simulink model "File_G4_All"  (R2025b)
settings: Solver=FixedStepDiscrete  StartTime=0.0  StopTime=inf  FixedStep=0.001  RelTol=1e-3  EnableMultiTasking=on
InitFcn:
  | np=4;
  | ke=0.035;
  | wn=4000/60*2*pi;
  | Tn=0.063; %Nm
  | B=Tn*0.1/wn;
  | inertia=2.4e-6; %kgm2
  | kfan=(Tn*0.9)/wn/wn;
undefined symbols (not defined in the file): DiscIntNeverNeededParam
libraries: mcbeeMathTransformLib x4, stm32f4xxblockslib x3, slpidlib x3, stm32g4xxblockslib x1, simulink x1

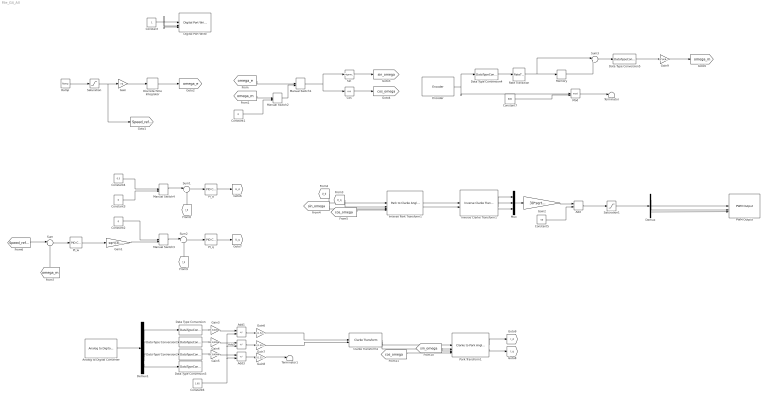
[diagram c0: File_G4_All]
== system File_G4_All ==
  Add : Sum
  Add1 : Sum  Inputs=+-
  Add2 : Sum  Inputs=+-
  Add3 : Sum  Inputs=+-
  Analog to Digital Converter : stm32f4xxblockslib/Analog to Digital Converter  ADCModule=ADC1  ConversionGroup=Injected  TriggerMode=Trigger and read  NumberOfConversions=4  EnableBufferConv=off  BufferLength=1  OutputStatus=off  SampleTime=-1  EnableSimPort=off  hoistedMaskSrc=ECSoC/ECSimCodegen/Analog to Digital Converter
  Clarke Transform1 : mcbeeMathTransformLib/Clarke Transform  VariantControl=Variant2  PowerInvariant=off  UseWithEmbedded=on  PhaseInput=Two inputs
  Constant : Constant
  Constant1 : Constant  Value=0
  Constant2 : Constant  Value=0
  Constant3 : Constant  Value=0
  Constant4 : Constant  Value=0.5
  Constant5 : Constant  Value=50
  Constant6 : Constant  Value=1.65
  Constant7 : Constant  Value=600  OutDataTypeStr=uint32
  Cos : Trigonometry  Operator=cos
  Data Type Conversion{,1..3,5} (5 alike) : DataTypeConversion  OutDataTypeStr=double
  Data Type Conversion4 : DataTypeConversion  OutDataTypeStr=int32
  Demux : Demux  Outputs=3
  Demux1 : Demux
  Digital Port Write : stm32f4xxblockslib/Digital Port Write  PortName=GPIOC  PinNumber=[10 11 12]  ReadOperation=off  IOAsArray=off  EnableSimPort=off  hoistedMaskSrc=ECSoC/ECSimCodegen/Digital Port Write
  Discrete-Time Integrator : DiscreteIntegrator  SampleTime=-1  ICPrevOutput=DiscIntNeverNeededParam  ICPrevScaledInput=DiscIntNeverNeededParam
  Encoder : stm32g4xxblockslib/Encoder  TimerModule=TIM2  EnableResetInput=off  OutputCountAfterFirstIndex=off  OutputValidIndex=off  OutputDirection=on  OutputStatus=off  SampleTime=-1
  Gain : Gain  Gain=np
  Gain1 : Gain  Gain=sqrt(3)/ke
  Gain2 : Gain  Gain=30*sqrt(2)/24
  Gain3 : Gain  Gain=3.3/4096
  Gain4 : Gain  Gain=3.3/4096
  Gain5 : Gain  Gain=3.3/4096
  Gain6 : Gain  Gain=1/(1.5278*0.33)
  Gain7 : Gain  Gain=1/(1.5278*0.33)
  Gain8 : Gain  Gain=1/(1.5278*0.33)
  Gain9 : Gain  Gain=(2*pi/600)/0.001
  Inverse Clarke Transform1 : mcbeeMathTransformLib/Inverse Clarke Transform  PowerInvariant=off  UseWithEmbedded=on  PhaseInput=Two inputs
  Inverse Park Transform1 : mcbeeMathTransformLib/Park to Clarke Angle Transform  AxisAlignment=D-axis  UseWithEmbedded=on  PhaseInput=Two inputs  ThetaInput=Sine and Cosine electrical position  AngleInput=Per-unit  N_points=1024
  Manual Switch1 : ManualSwitch  CurrentSetting=0
  Manual Switch2 : ManualSwitch  CurrentSetting=0
  Manual Switch3 : ManualSwitch
  Manual Switch4 : ManualSwitch
  Memory : Memory
  Mod : Math  Operator=mod
  Mux : Mux  Inputs=3
  PI_d : slpidlib/PID Controller  Controller=PI  Form=Parallel  TimeDomain=Discrete-time  UseExternalTs=off  SampleTime=-1  IntegratorMethod=Forward Euler  FilterMethod=Forward Euler  ControllerParametersSource=internal  P=23.334  I=16666.67  UseKiTs=off  D=0  UseExternalDerivativeSource=off  N=100  UseFilter=on  TunerSelectOption=Transfer Function Based (PID Tuner App)  InitialConditionSource=internal  InitialConditionForIntegrator=0  InitialConditionForFilter=0  DifferentiatorICPrevScaledInput=0  ExternalReset=none  TrackingMode=off  Kt=1  LimitOutput=off  SatLimitsSource=internal  UpperSaturationLimit=inf  LowerSaturationLimit=-inf  LinearizeAsGain=on  AntiWindupMode=none  Kb=1  LimitIntegrator=off  UpperIntegratorSaturationLimit=inf  LowerIntegratorSaturationLimit=-inf  POutMin=[]  POutMax=[]  IOutMin=[]  IOutMax=[]  DOutMin=[]  DOutMax=[]  NOutMin=[]  NOutMax=[]  SumOutMin=[]  SumOutMax=[]  SaturationOutMin=[]  SaturationOutMax=[]  PParamMin=[]  PParamMax=[]  IParamMin=[]  IParamMax=[]  DParamMin=[]  DParamMax=[]  NParamMin=[]  NParamMax=[]  KbParamMin=[]  KbParamMax=[]  KtParamMin=[]  KtParamMax=[]  KbOutMin=[]  KbOutMax=[]  KtOutMin=[]  KtOutMax=[]  IntegratorOutMin=[]  IntegratorOutMax=[]  FilterOutMin=[]  FilterOutMax=[]  SumI1OutMin=[]  SumI1OutMax=[]  SumI2OutMin=[]  SumI2OutMax=[]  SumI3OutMin=[]  SumI3OutMax=[]  SumI4OutMin=[]  SumI4OutMax=[]  SumDOutMin=[]  SumDOutMax=[]  DifferentiatorOutMin=[]  DifferentiatorOutMax=[]  FilterDiffOutCoefMin=[]  FilterDiffOutCoefMax=[]  ReciprocalOutMin=[]  ReciprocalOutMax=[]  SumDenOutMin=[]  SumDenOutMax=[]  SumNumOutMin=[]  SumNumOutMax=[]  DivideOutMin=[]  DivideOutMax=[]  UdiffTsProdOutMin=[]  UdiffTsProdOutMax=[]  NTsProdOutMin=[]  NTsProdOutMax=[]  UintegralTsProdOutMin=[]  UintegralTsProdOutMax=[]  UngainTsProdOutMin=[]  UngainTsProdOutMax=[]  ClampingZeroOutDataTypeStr=Inherit: Inherit via back propagation  ClampingZeroOutMin=[]  ClampingZeroOutMax=[]  FilterDenConstantOutDataTypeStr=Inherit: Inherit via back propagation  FilterDenConstantOutMin=[]  FilterDenConstantOutMax=[]  PCopyOutDataTypeStr=Inherit: Inherit via back propagation  PCopyOutMin=[]  PCopyOutMax=[]  NCopyOutDataTypeStr=Inherit: Inherit via back propagation  NCopyOutMin=[]  NCopyOutMax=[]  IntegratorContinuousStateAttributes=''  IntegratorStateMustResolveToSignalObject=off  IntegratorRTWStateStorageClass=Auto  FilterContinuousStateAttributes=''  FilterStateMustResolveToSignalObject=off  FilterRTWStateStorageClass=Auto  ParallelPVariant=InternalParameters  IdealPVariant=Disabled  IVariant=InternalParameters  DVariant=Disabled  IntegratorVariant=Discrete  SatVariant=Disabled  AWVariant=Passthrough  PCopyVariant=Disabled  TRVariant=Disabled  FdbkBlocksVariant=Forward  IdealPFdbkVariant=Disabled  SatFdbkVariant=Disabled  DerivativeFilterVariant=Disabled  NVariant=Disabled  NCopyVariant=Disabled_SignalSpec  FilterICVariant=Disabled  IntegratorICVariant=InternalICs  ExternalResetVariant=Disabled  TRSumVariant=Passthrough  SumFdbkVariant=Disabled  SumVariant=Sum_PI  TsampFilterVariant=InternalTs  TsampNgainVariant=Passthrough  TsampIntegralVariant=Disabled_SignalSpec  ExternalSaturationOutDataTypeStr=Inherit: Same as second input  DerivativeSourceVariant=Disabled  PreIntVariant=InternalPreInt
  PI_q : slpidlib/PID Controller  Controller=PI  Form=Parallel  TimeDomain=Discrete-time  UseExternalTs=off  SampleTime=-1  IntegratorMethod=Forward Euler  FilterMethod=Forward Euler  ControllerParametersSource=internal  P=23.334  I=16666.67  UseKiTs=off  D=0  UseExternalDerivativeSource=off  N=100  UseFilter=on  TunerSelectOption=Transfer Function Based (PID Tuner App)  InitialConditionSource=internal  InitialConditionForIntegrator=0  InitialConditionForFilter=0  DifferentiatorICPrevScaledInput=0  ExternalReset=none  TrackingMode=off  Kt=1  LimitOutput=off  SatLimitsSource=internal  UpperSaturationLimit=inf  LowerSaturationLimit=-inf  LinearizeAsGain=on  AntiWindupMode=none  Kb=1  LimitIntegrator=off  UpperIntegratorSaturationLimit=inf  LowerIntegratorSaturationLimit=-inf  POutMin=[]  POutMax=[]  IOutMin=[]  IOutMax=[]  DOutMin=[]  DOutMax=[]  NOutMin=[]  NOutMax=[]  SumOutMin=[]  SumOutMax=[]  SaturationOutMin=[]  SaturationOutMax=[]  PParamMin=[]  PParamMax=[]  IParamMin=[]  IParamMax=[]  DParamMin=[]  DParamMax=[]  NParamMin=[]  NParamMax=[]  KbParamMin=[]  KbParamMax=[]  KtParamMin=[]  KtParamMax=[]  KbOutMin=[]  KbOutMax=[]  KtOutMin=[]  KtOutMax=[]  IntegratorOutMin=[]  IntegratorOutMax=[]  FilterOutMin=[]  FilterOutMax=[]  SumI1OutMin=[]  SumI1OutMax=[]  SumI2OutMin=[]  SumI2OutMax=[]  SumI3OutMin=[]  SumI3OutMax=[]  SumI4OutMin=[]  SumI4OutMax=[]  SumDOutMin=[]  SumDOutMax=[]  DifferentiatorOutMin=[]  DifferentiatorOutMax=[]  FilterDiffOutCoefMin=[]  FilterDiffOutCoefMax=[]  ReciprocalOutMin=[]  ReciprocalOutMax=[]  SumDenOutMin=[]  SumDenOutMax=[]  SumNumOutMin=[]  SumNumOutMax=[]  DivideOutMin=[]  DivideOutMax=[]  UdiffTsProdOutMin=[]  UdiffTsProdOutMax=[]  NTsProdOutMin=[]  NTsProdOutMax=[]  UintegralTsProdOutMin=[]  UintegralTsProdOutMax=[]  UngainTsProdOutMin=[]  UngainTsProdOutMax=[]  ClampingZeroOutDataTypeStr=Inherit: Inherit via back propagation  ClampingZeroOutMin=[]  ClampingZeroOutMax=[]  FilterDenConstantOutDataTypeStr=Inherit: Inherit via back propagation  FilterDenConstantOutMin=[]  FilterDenConstantOutMax=[]  PCopyOutDataTypeStr=Inherit: Inherit via back propagation  PCopyOutMin=[]  PCopyOutMax=[]  NCopyOutDataTypeStr=Inherit: Inherit via back propagation  NCopyOutMin=[]  NCopyOutMax=[]  IntegratorContinuousStateAttributes=''  IntegratorStateMustResolveToSignalObject=off  IntegratorRTWStateStorageClass=Auto  FilterContinuousStateAttributes=''  FilterStateMustResolveToSignalObject=off  FilterRTWStateStorageClass=Auto  ParallelPVariant=InternalParameters  IdealPVariant=Disabled  IVariant=InternalParameters  DVariant=Disabled  IntegratorVariant=Discrete  SatVariant=Disabled  AWVariant=Passthrough  PCopyVariant=Disabled  TRVariant=Disabled  FdbkBlocksVariant=Forward  IdealPFdbkVariant=Disabled  SatFdbkVariant=Disabled  DerivativeFilterVariant=Disabled  NVariant=Disabled  NCopyVariant=Disabled_SignalSpec  FilterICVariant=Disabled  IntegratorICVariant=InternalICs  ExternalResetVariant=Disabled  TRSumVariant=Passthrough  SumFdbkVariant=Disabled  SumVariant=Sum_PI  TsampFilterVariant=InternalTs  TsampNgainVariant=Passthrough  TsampIntegralVariant=Disabled_SignalSpec  ExternalSaturationOutDataTypeStr=Inherit: Same as second input  DerivativeSourceVariant=Disabled  PreIntVariant=InternalPreInt
  PI_w : slpidlib/PID Controller  Controller=PI  Form=Parallel  TimeDomain=Discrete-time  UseExternalTs=off  SampleTime=-1  IntegratorMethod=Forward Euler  FilterMethod=Forward Euler  ControllerParametersSource=internal  P=0.087703  I=1.7994  UseKiTs=off  D=0  UseExternalDerivativeSource=off  N=100  UseFilter=on  TunerSelectOption=Transfer Function Based (PID Tuner App)  InitialConditionSource=internal  InitialConditionForIntegrator=0  InitialConditionForFilter=0  DifferentiatorICPrevScaledInput=0  ExternalReset=none  TrackingMode=off  Kt=1  LimitOutput=off  SatLimitsSource=internal  UpperSaturationLimit=inf  LowerSaturationLimit=-inf  LinearizeAsGain=on  AntiWindupMode=none  Kb=1  LimitIntegrator=off  UpperIntegratorSaturationLimit=inf  LowerIntegratorSaturationLimit=-inf  POutMin=[]  POutMax=[]  IOutMin=[]  IOutMax=[]  DOutMin=[]  DOutMax=[]  NOutMin=[]  NOutMax=[]  SumOutMin=[]  SumOutMax=[]  SaturationOutMin=[]  SaturationOutMax=[]  PParamMin=[]  PParamMax=[]  IParamMin=[]  IParamMax=[]  DParamMin=[]  DParamMax=[]  NParamMin=[]  NParamMax=[]  KbParamMin=[]  KbParamMax=[]  KtParamMin=[]  KtParamMax=[]  KbOutMin=[]  KbOutMax=[]  KtOutMin=[]  KtOutMax=[]  IntegratorOutMin=[]  IntegratorOutMax=[]  FilterOutMin=[]  FilterOutMax=[]  SumI1OutMin=[]  SumI1OutMax=[]  SumI2OutMin=[]  SumI2OutMax=[]  SumI3OutMin=[]  SumI3OutMax=[]  SumI4OutMin=[]  SumI4OutMax=[]  SumDOutMin=[]  SumDOutMax=[]  DifferentiatorOutMin=[]  DifferentiatorOutMax=[]  FilterDiffOutCoefMin=[]  FilterDiffOutCoefMax=[]  ReciprocalOutMin=[]  ReciprocalOutMax=[]  SumDenOutMin=[]  SumDenOutMax=[]  SumNumOutMin=[]  SumNumOutMax=[]  DivideOutMin=[]  DivideOutMax=[]  UdiffTsProdOutMin=[]  UdiffTsProdOutMax=[]  NTsProdOutMin=[]  NTsProdOutMax=[]  UintegralTsProdOutMin=[]  UintegralTsProdOutMax=[]  UngainTsProdOutMin=[]  UngainTsProdOutMax=[]  ClampingZeroOutDataTypeStr=Inherit: Inherit via back propagation  ClampingZeroOutMin=[]  ClampingZeroOutMax=[]  FilterDenConstantOutDataTypeStr=Inherit: Inherit via back propagation  FilterDenConstantOutMin=[]  FilterDenConstantOutMax=[]  PCopyOutDataTypeStr=Inherit: Inherit via back propagation  PCopyOutMin=[]  PCopyOutMax=[]  NCopyOutDataTypeStr=Inherit: Inherit via back propagation  NCopyOutMin=[]  NCopyOutMax=[]  IntegratorContinuousStateAttributes=''  IntegratorStateMustResolveToSignalObject=off  IntegratorRTWStateStorageClass=Auto  FilterContinuousStateAttributes=''  FilterStateMustResolveToSignalObject=off  FilterRTWStateStorageClass=Auto  ParallelPVariant=InternalParameters  IdealPVariant=Disabled  IVariant=InternalParameters  DVariant=Disabled  IntegratorVariant=Discrete  SatVariant=Disabled  AWVariant=Passthrough  PCopyVariant=Disabled  TRVariant=Disabled  FdbkBlocksVariant=Forward  IdealPFdbkVariant=Disabled  SatFdbkVariant=Disabled  DerivativeFilterVariant=Disabled  NVariant=Disabled  NCopyVariant=Disabled_SignalSpec  FilterICVariant=Disabled  IntegratorICVariant=InternalICs  ExternalResetVariant=Disabled  TRSumVariant=Passthrough  SumFdbkVariant=Disabled  SumVariant=Sum_PI  TsampFilterVariant=InternalTs  TsampNgainVariant=Passthrough  TsampIntegralVariant=Disabled_SignalSpec  ExternalSaturationOutDataTypeStr=Inherit: Same as second input  DerivativeSourceVariant=Disabled  PreIntVariant=InternalPreInt
  PWM Output : stm32f4xxblockslib/PWM Output  ProcessorFamily=STM32G4  TimerModule=TIM1  DutycycleUnits=Percentage  EnableChannel1=on  EnableCaptureCompare1Input=off  EnableCaptureCompare1ComplementaryInput=off  EnableOutputCompare1ModeInput=off  EnableChannel2=on  EnableCaptureCompare2Input=off  EnableCaptureCompare2ComplementaryInput=off  EnableOutputCompare2ModeInput=off  EnableChannel3=on  EnableCaptureCompare3Input=off  EnableCaptureCompare3ComplementaryInput=off  EnableOutputCompare3ModeInput=off  EnableChannel4=off  EnableCaptureCompare4Input=off  EnableCaptureCompare4ComplementaryInput=off  EnableOutputCompare4ModeInput=off  EnableChannel5=off  EnableCaptureCompare5Input=off  EnableOutputCompare5ModeInput=off  EnableChannel6=off  EnableCaptureCompare6Input=off  EnableOutputCompare6ModeInput=off  EnableCounterInput=off  EnableMainOutputInput=off  EnableFrequencyInput=off  SetRCAfterCE=off  OutputDirection=off  OutputMainOutputEnableStatus=off  SampleTime=0.1  EnableSimPort=off  EnableUpdateEvent=off  EnableCaptureCompare1Event=off  EnableCaptureCompare2Event=off  EnableCaptureCompare3Event=off  EnableCaptureCompare4Event=off  EnableTriggerEvent=off  EnableBreakEvent=off  EnableBreakEvent2=off  hoistedMaskSrc=ECSoC/ECSimCodegen/PWM Output
  Park Transform1 : mcbeeMathTransformLib/Clarke to Park Angle Transform  AxisAlignment=D-axis  UseWithEmbedded=on  PhaseInput=Two inputs  ThetaInput=Sine and Cosine electrical position  AngleInput=Per-unit  N_points=1024
  Ramp : simulink/Sources/Ramp  slope=wn/4  start=0  InitialOutput=0
  Rate Transition : RateTransition  OutPortSampleTime=0.001
  Saturation : Saturate  UpperLimit=wn  LowerLimit=0
  Saturation1 : Saturate  UpperLimit=80  LowerLimit=20
  Sin : Trigonometry
  Sum : Sum  Inputs=|+-
  Sum1 : Sum  Inputs=|++
  Sum2 : Sum  Inputs=|++
  Sum3 : Sum  Inputs=|+-
  Terminator : Terminator
  Terminator1 : Terminator
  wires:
  Ramp/1 -> Saturation/1
  Saturation/1 -> [Speed_ref_e], Gain/1
  Gain/1 -> Discrete-Time Integrator/1
  Sin/1 -> [sin_omega]
  Cos/1 -> [cos_omega]
  Manual Switch1/1 -> Sin/1, Cos/1
  [omega_e] -> Manual Switch1/1
  Manual Switch2/1 -> Manual Switch1/2
  [omega_m] -> Manual Switch2/1
  Constant1/1 -> Manual Switch2/2
  [sin_omega] -> Inverse Park Transform1/3
  [cos_omega] -> Inverse Park Transform1/4
  Inverse Park Transform1/1 -> Inverse Clarke Transform1/1
  Inverse Park Transform1/2 -> Inverse Clarke Transform1/2
  [Speed_ref_e] -> Sum/1
  Sum/1 -> PI_w/1
  [omega_m] -> Sum/2
  PI_w/1 -> Gain1/1
  Gain1/1 -> Manual Switch3/2
  Manual Switch3/1 -> Sum2/1
  Constant2/1 -> Manual Switch3/1
  Constant3/1 -> Manual Switch4/2
  Constant4/1 -> Manual Switch4/1
  Manual Switch4/1 -> Sum1/1
  Sum1/1 -> PI_d/1
  PI_d/1 -> [U_d]
  PI_q/1 -> [U_q]
  Sum2/1 -> PI_q/1
  [U_q] -> Inverse Park Transform1/2
  [U_d] -> Inverse Park Transform1/1
  [I_d] -> Sum1/2
  [I_q] -> Sum2/2
  Clarke Transform1/2 -> Park Transform1/2
  Clarke Transform1/1 -> Park Transform1/1
  Park Transform1/1 -> [I_d]
  Park Transform1/2 -> [I_q]
  [sin_omega] -> Park Transform1/3
  [cos_omega] -> Park Transform1/4
  Constant/1 -> Digital Port Write/3, Digital Port Write/1, Digital Port Write/2
  Inverse Clarke Transform1/3 -> Mux/3
  Inverse Clarke Transform1/2 -> Mux/2
  Inverse Clarke Transform1/1 -> Mux/1
  Mux/1 -> Gain2/1
  Demux/2 -> PWM Output/2
  Demux/1 -> PWM Output/1
  Demux/3 -> PWM Output/3
  Add/1 -> Saturation1/1
  Gain2/1 -> Add/1
  Constant5/1 -> Add/2
  Saturation1/1 -> Demux/1
  Demux1/1 -> Data Type Conversion/1
  Demux1/2 -> Data Type Conversion1/1
  Demux1/3 -> Data Type Conversion2/1
  Demux1/4 -> Data Type Conversion3/1
  Data Type Conversion/1 -> Gain3/1
  Gain3/1 -> Add1/1
  Add1/1 -> Gain6/1
  Add2/1 -> Gain7/1
  Add3/1 -> Gain8/1
  Data Type Conversion1/1 -> Gain4/1
  Data Type Conversion2/1 -> Gain5/1
  Gain4/1 -> Add2/1
  Gain5/1 -> Add3/1
  Constant6/1 -> Add3/2, Add2/2, Add1/2
  Gain6/1 -> Clarke Transform1/1
  Gain7/1 -> Clarke Transform1/2
  Encoder/1 -> Data Type Conversion4/1, Mod/1
  Data Type Conversion4/1 -> Rate Transition/1
  Rate Transition/1 -> Sum3/1, Memory/1
  Memory/1 -> Sum3/2
  Sum3/1 -> Data Type Conversion5/1
  Data Type Conversion5/1 -> Gain9/1
  Gain9/1 -> [omega_m]
  Constant7/1 -> Mod/2
  Mod/1 -> Terminator/1
  Gain8/1 -> Terminator1/1
  Analog to Digital Converter/1 -> Demux1/1
  Discrete-Time Integrator/1 -> [omega_e]
